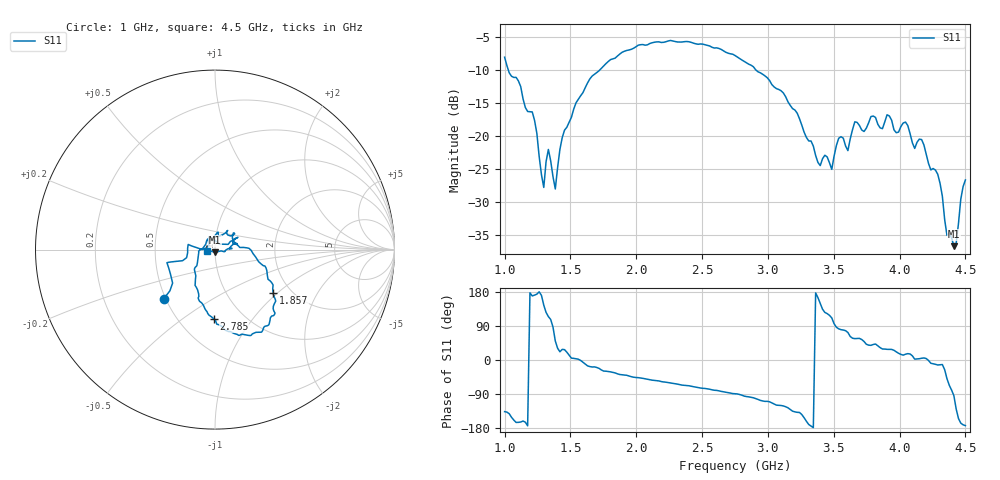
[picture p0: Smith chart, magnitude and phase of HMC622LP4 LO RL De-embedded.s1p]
! Hittite Microwave Corporation
! 20 Alpha Road
! Chelmsford, MA 01824
! http://www.hittite.com
! Tel: 978-250-3343
! Fax: 978-250-3373
! Device:  HMC622LP4
! Description:  GaAS MMIC MIXER With integrated IF/LO Amplifier
! Frequency:  1.8-  3.9 GHz
! Package:
! Data:  The device was measured on evaluation board 119242
!  The evaluation circuit board was modeled and simulated.  This was use
!  to removed the evaluation board circuit from the measured data.
!  The reference plane is the center of the package pin.
! Misc:
! Date Measured:  06-09-2009
! Date:  08-24-2009
! Note:
!  Hittite supplies this data as a sample of measured data at the package pin for
!  for this package product.  Your particular data for this product may vary.
!  Data was taken at 25 degrees C.
!  Hittite reserves the right to change this data at anytime
# MHz S MA R 50
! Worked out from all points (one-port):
!   201 points, 1 GHz to 4.5 GHz, reference 50 ohm
!   lowest |S11| = -36.7 dB at 4.412 GHz (marker M1), VSWR 1.03, Z = 49.9 - j1.46 ohm
!   |S11| at or under -10 dB: 1.028 GHz to 1.723 GHz (695.4 MHz wide, 50.6 % of centre); 2.908 GHz to end of sweep
!   S11 on the Smith chart (normalised r, x): 1 GHz: 0.49, -0.32; 1.857 GHz: 1.63, -0.93; 2.785 GHz: 0.73, -0.66; 4.5 GHz: 0.91, -0.01
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1000  0.3944 -136.2
1210  0.1521 169.1
1297.5  0.04086 144.7
1332.5  0.07916 114.5
1385  0.03975 50.2
1437.5  0.09711 28.0
1647.5  0.2703 -17.4
1857.5  0.403 -36.6
1875  0.4168 -38.3
2312.5  0.5144 -63.6
2750  0.4064 -89.1
2785  0.3855 -91.0
3187.5  0.1612 -135.1
3397.5  0.05977 149.2
3432.5  0.07154 125.6
3485  0.05596 111.1
3537.5  0.0961 82.2
3607.5  0.07756 72.6
3625  0.09496 62.2
3660  0.1281 56.4
3730  0.1082 48.9
3800  0.1416 41.0
4062.5  0.12 16.8
4115  0.08054 2.3
4290  0.05139 -13.1
4360  0.01773 -49.2
4412.5  0.01469 -93.9
4500  0.04654 -173.2
